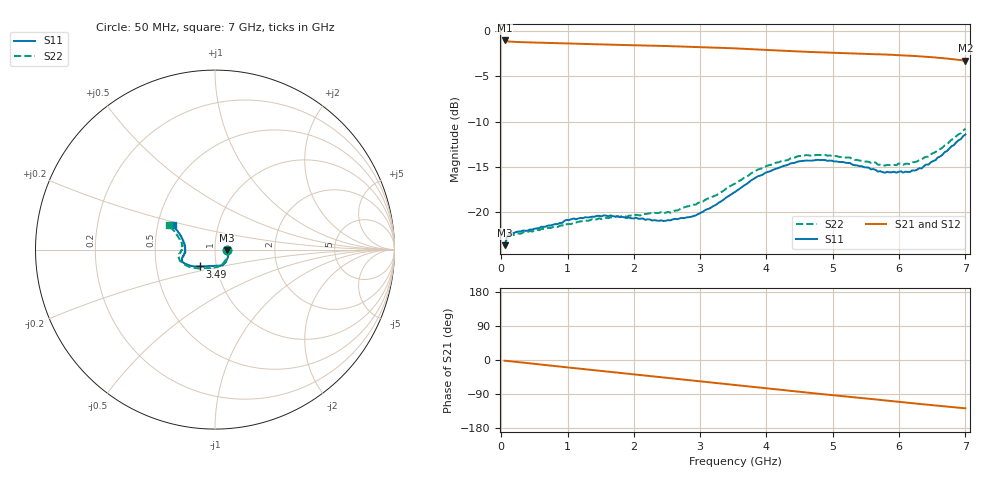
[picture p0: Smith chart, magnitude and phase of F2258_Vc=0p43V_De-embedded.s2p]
! Integrated Device Technology
! Corporate Headquarters
! 6024 Silver Creek Valley Road
! San Jose, CA 95138  USA
! Phone:  1-408-284-8200
! Toll Free:  1-800-223-1366
! Webpage:  http://www.idt.com/
! Timing and RF Division
! 515 Groton Road, Suite 102
! Westford, MA 01886-6024
! Device:  F2258
! Description: Voltage Variable RF Attenuator
! Frequency:  50.0 -  6000.00 MHz
! Package:  3x3 mm Thin QFN Plastic Package: 16 pin
! Ports:  2 RF, 2 DC
!  Pin  1  = NC
!  Pin  2  = NC
!  Pin  3  = RF2  = Port 2
!  Pin  4  = GND
!  Pin  5  = Vdd
!  Pin  6  = NC
!  Pin  7  = VCTRL
!  Pin  8  = NC
!  Pin  9  = GND
!  Pin 10  = RF1  = Port 1
!  Pin 11  = NC
!  Pin 12  = NC
!  Pin 13  = NC
!  Pin 14  = NC
!  Pin 15  = NC
!  Pin 16  = NC
! Vcntrl:  0.430 Volts
! Vdd:  +3.300 Volts
! Current:  1.097 mA
! Data:  The device was measured on a the F2258 evaluation board which has
!  individual transmission lines to the RF pins.  Data was collected
!  using a calibrated network analyzer.  The evaluation board was
!  de-embedded using a TRL calibration technique.
!  The reference plane is the edge of the package pin.
! Misc:  SN 10
!  Action Tracker AT0285
! Date Measured:  2014-12-10
! Date:  2016-01-13  MJV
! Note:
!  Integrated Device Technology supplies this data as a sample of measured
!  data at the package pin for this product.  Your particular data for this
!  product may vary.
!  Data was taken at 25 degrees C.
!  Integrated Device Technology reserves the right to change this data at anytime.
!Freq_(GHz)  S11M_(dB)  S11P_(deg)  S21M_(dB)  S21P_(deg)  S12M_(dB)  S12P_(deg)  S22M_(dB)  S22P_(deg)
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# GHz S dB R 50
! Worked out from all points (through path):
!   201 points, 50 MHz to 7 GHz, reference 50 ohm
!   highest |S21| = -1.04 dB at 50 MHz (marker M1); lowest = -3.3 dB at 7 GHz (marker M2)
!   group delay of S21, straight-line fit = 50.5 ps
!   lowest |S11| = -23.7 dB at 50 MHz (marker M3), VSWR 1.14, Z = 57 - j0.433 ohm
!   |S11| at or under -10 dB: start of sweep to end of sweep
!   |S22| runs from -23.8 to -10.8 dB; largest |S21 - S12| = 0.00034
!   S11 on the Smith chart (normalised r, x): 50 MHz: 1.14, -0.01; 3.49 GHz: 0.83, -0.16; 7 GHz: 0.60, +0.18
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0.05  -23.67 -3.3  -1.04 -2.0  -1.04 -2.0  -23.75 -3.0
0.08475  -22.75 -5.3  -1.12 -2.5  -1.12 -2.5  -22.85 -5.2
0.15425  -22.28 -8.3  -1.18 -3.6  -1.18 -3.7  -22.49 -8.9
0.71025  -21.47 -34.0  -1.31 -14.1  -1.31 -14.1  -21.72 -36.7
0.98825  -20.84 -47.1  -1.36 -19.4  -1.36 -19.4  -21.32 -52.1
1.2315  -20.66 -55.0  -1.42 -23.8  -1.42 -23.8  -21.00 -61.0
1.6485  -20.36 -66.4  -1.50 -31.4  -1.50 -31.4  -20.57 -74.1
2.37825  -20.95 -86.7  -1.63 -44.8  -1.63 -44.8  -20.08 -92.2
2.552  -20.91 -92.5  -1.67 -48.0  -1.67 -48.0  -20.06 -97.6
2.93425  -20.35 -109.2  -1.75 -55.1  -1.75 -55.1  -19.16 -111.1
3.49025  -17.92 -132.5  -1.90 -65.6  -1.90 -65.6  -16.97 -132.6
3.525  -17.77 -133.4  -1.91 -66.2  -1.91 -66.2  -16.84 -134.1
4.0115  -15.57 -148.1  -2.09 -75.2  -2.09 -75.2  -14.86 -149.8
4.46325  -14.43 -156.9  -2.25 -83.4  -2.25 -83.4  -13.85 -161.1
4.7065  -14.29 -160.2  -2.32 -87.7  -2.32 -87.7  -13.74 -165.4
5.2625  -14.58 -167.0  -2.48 -97.4  -2.48 -97.4  -13.97 -173.6
5.6795  -15.52 -173.5  -2.56 -104.6  -2.56 -104.6  -14.76 -179.1
5.85325  -15.60 -177.7  -2.61 -107.8  -2.62 -107.8  -14.79 176.2
6.166  -15.56 174.3  -2.72 -113.4  -2.72 -113.4  -14.71 170.2
6.33975  -15.17 167.8  -2.80 -116.5  -2.80 -116.5  -14.19 165.8
6.722  -13.25 155.4  -3.04 -123.1  -3.04 -123.1  -12.54 156.6
7  -11.41 149.6  -3.28 -127.4  -3.28 -127.4  -10.79 151.7
